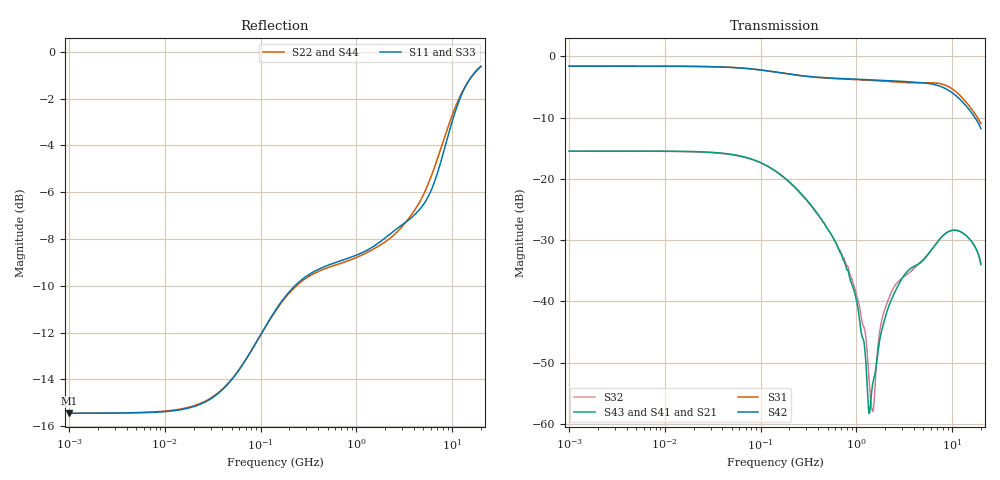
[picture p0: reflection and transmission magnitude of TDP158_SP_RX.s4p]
! Created Wed Jun 08 14:21:48 2016
# hz S db R 50
! 4 Port Network Data from SP1.SP block
! freq  dbS11  angS11  dbS12  angS12  dbS13  angS13  dbS14  angS14
!  dbS21  angS21  dbS22  angS22  dbS23  angS23  dbS24  angS24
!  dbS31  angS31  dbS32  angS32  dbS33  angS33  dbS34  angS34
!  dbS41  angS41  dbS42  angS42  dbS43  angS43  dbS44  angS44
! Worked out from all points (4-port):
!   861 points, 1 MHz to 20 GHz, reference 50 ohm
!   strongest paths, dB at 1 MHz, 11.89 MHz, 141.4 MHz, 1.682 GHz, 20 GHz:
!     S42: -1.6, -1.6, -2.6, -3.9, -11.8
!     S31: -1.6, -1.6, -2.6, -4.0, -11.0
!     S43: -15.5, -15.5, -18.6, -48.2, -33.9
!     S41: -15.5, -15.5, -18.6, -48.2, -33.9
!     S21: -15.5, -15.5, -18.6, -48.2, -33.9
!     S32: -15.5, -15.5, -18.7, -47.2, -34.0
!   lowest |S11| = -15.4 dB at 1 MHz (marker M1), VSWR 1.41, Z = 35.5 - j0.101 ohm
!   |S11| at or under -10 dB: start of sweep to 228 MHz
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1000000  -15.45 -179.5  -15.48 -0.4  -1.61 -0.1  -15.48 -0.4
         -15.48 -0.4  -15.44 -179.5  -15.48 -0.4  -1.61 -0.1
         -1.61 -0.1  -15.48 -0.4  -15.45 -179.5  -15.48 -0.4
         -15.48 -0.4  -1.61 -0.1  -15.48 -0.4  -15.44 -179.5
1.80111e8  -10.47 -160.9  -19.97 -56.2  -2.81 -7.8  -19.97 -56.2
           -19.88 -56.3  -10.52 -161.2  -19.88 -56.3  -2.80 -7.6
           -2.81 -7.8  -19.97 -56.2  -10.47 -160.9  -19.97 -56.2
           -19.88 -56.3  -2.80 -7.6  -19.88 -56.3  -10.52 -161.2
8.427536e8  -8.80 -167.7  -35.15 -99.5  -3.74 -6.8  -35.15 -99.5
            -35.78 -101.7  -8.91 -167.5  -35.78 -101.7  -3.68 -6.8
            -3.74 -6.8  -35.15 -99.5  -8.80 -167.7  -35.15 -99.5
            -35.78 -101.7  -3.68 -6.8  -35.78 -101.7  -8.91 -167.5
1.464732e9  -8.35 -165.5  -57.69 146.3  -3.92 -8.6  -57.69 146.3
            -54.01 94.8  -8.46 -165.2  -54.01 94.8  -3.85 -8.6
            -3.92 -8.6  -57.69 146.3  -8.35 -165.5  -57.69 146.3
            -54.01 94.8  -3.85 -8.6  -54.01 94.8  -8.46 -165.2
2.605062e9  -7.58 -162.1  -37.13 43.4  -4.21 -12.0  -37.13 43.4
            -38.03 46.8  -7.74 -160.3  -38.03 46.8  -4.03 -12.7
            -4.21 -12.0  -37.13 43.4  -7.58 -162.1  -37.13 43.4
            -38.03 46.8  -4.03 -12.7  -38.03 46.8  -7.74 -160.3
9.681765e9  -3.19 -148.0  -28.44 3.8  -5.16 -41.7  -28.44 3.8
            -28.46 3.8  -2.88 -150.6  -28.46 3.8  -5.77 -43.2
            -5.16 -41.7  -28.44 3.8  -3.19 -148.0  -28.44 3.8
            -28.46 3.8  -5.77 -43.2  -28.46 3.8  -2.88 -150.6
2e10  -0.62 -163.6  -33.98 -41.2  -10.96 -68.0  -33.98 -41.2
      -33.95 -41.2  -0.64 -165.3  -33.95 -41.2  -11.79 -66.7
      -10.96 -68.0  -33.98 -41.2  -0.62 -163.6  -33.98 -41.2
      -33.95 -41.2  -11.79 -66.7  -33.95 -41.2  -0.64 -165.3
